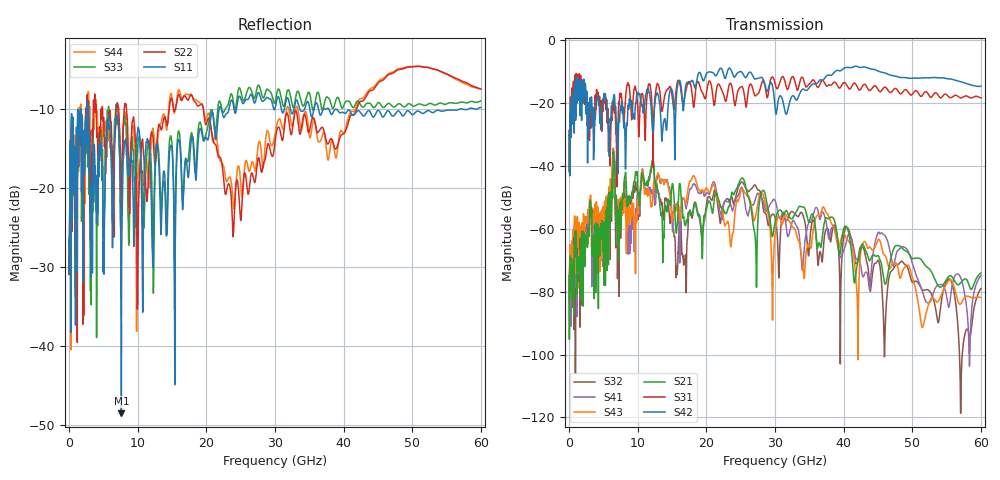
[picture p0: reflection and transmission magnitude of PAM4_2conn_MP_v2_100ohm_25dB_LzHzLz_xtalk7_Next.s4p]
! Info: Touchstone file created by Circ.  Input file=FAB50GbE_2conn_Midplane_Examax_Topo2_v2_100ohm_25dB_LzHzLz.circ
# Hz S RI R 50
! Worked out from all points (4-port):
!   6000 points, 10 MHz to 60 GHz, reference 50 ohm
!   strongest paths, dB at 10 MHz, 15.01 GHz, 30.01 GHz, 45.01 GHz, 60 GHz:
!     S42: -41.8, -15.8, -21.2, -9.7, -14.6
!     S31: -41.6, -17.8, -13.7, -15.6, -18.3
!     S21: -75.8, -45.9, -57.9, -68.5, -74.0
!     S43: -77.5, -56.2, -61.8, -63.5, -81.9
!     S41: -89.0, -56.9, -50.9, -61.2, -74.9
!     S32: -81.0, -56.3, -56.3, -70.0, -79.0
!   lowest |S11| = -48.5 dB at 7.62 GHz (marker M1), VSWR 1.01, Z = 50.4 + j0.119 ohm
!   |S11| at or under -10 dB: start of sweep to 1.262 GHz; 2.805 GHz to 21.85 GHz (19.05 GHz wide, 154 % of centre); 39 GHz to 56.78 GHz (17.78 GHz wide, 37.1 % of centre)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
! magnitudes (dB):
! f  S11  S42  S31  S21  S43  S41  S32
! 10 MHz  -30.9  -41.8  -41.6  -75.8  -77.5  -89.0  -81.0
! 1.28 GHz  -10.1  -12.0  -10.9  -69.4  -60.9  -63.7  -64.6
! 7.62 GHz  -48.5  -21.2  -17.3  -50.7  -50.1  -50.4  -50.3
! 12.12 GHz  -27.7  -27.5  -23.1  -38.2  -52.1  -48.9  -39.4
! 16.83 GHz  -17.3  -17.5  -18.3  -58.4  -51.1  -50.9  -69.8
! 25.21 GHz  -9.1  -10.2  -14.7  -43.8  -47.2  -46.9  -45.1
! 60 GHz  -9.7  -14.6  -18.3  -74.0  -81.9  -74.9  -79.0
